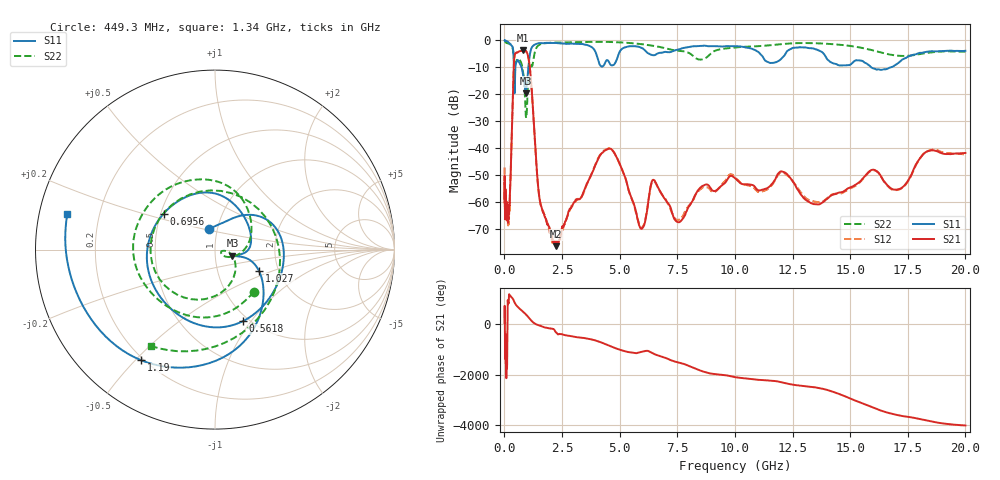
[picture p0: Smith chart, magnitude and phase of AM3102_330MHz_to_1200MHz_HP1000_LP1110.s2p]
! Date/Time: Tue, Sep 11, 2018 5:17 PM
! Network Analyzer: Agilent Technologies E8362B Rev: A.07.50.63
! Sweep from 0.010 to 20.000 GHz, 1601 Points, Sweep Type: LOG
! Power Supply: 4.949 V, 0.001 A
# Hz S DB R 50
!freq MagS11 AngS11 MagS21 AngS21 MagS12 AngS12 MagS22 AngS22
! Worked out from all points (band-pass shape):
!   1601 points, 10 MHz to 20 GHz, reference 50 ohm
!   highest |S21| = -3.57 dB at 813.7 MHz (marker M1); lowest = -76.5 dB at 2.249 GHz (marker M2)
!   |S21| within 3 dB of the highest: 429.5 MHz to 1.046 GHz (616.7 MHz wide, 83.6 % of centre)
!   lowest |S11| = -19.7 dB at 925.1 MHz (marker M3), VSWR 1.23, Z = 60.6 - j4.18 ohm
!   |S11| at or under -10 dB: 413.3 MHz to 476.9 MHz (63.61 MHz wide, 14.3 % of centre); 746.9 MHz to 1.041 GHz (294.2 MHz wide, 32.9 % of centre); 15.91 GHz to 16.77 GHz (858.9 MHz wide, 5.26 % of centre)
!   |S22| runs from -28.8 to -0.2 dB; largest |S21 - S12| = 0.0093
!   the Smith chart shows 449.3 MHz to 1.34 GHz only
!   S11 on the Smith chart (normalised r, x): 449.3 MHz: 0.91, +0.21; 561.8 MHz: 0.94, -0.91; 695.6 MHz: 0.52, +0.24; 1.027 GHz: 1.59, -0.41; 1.19 GHz: 0.19, -0.52; 1.34 GHz: 0.08, +0.12
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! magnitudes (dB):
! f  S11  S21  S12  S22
! 10 MHz  0.0  -51.9  -47.3  -0.3
! 35.55 MHz  0.0  -63.0  -63.6  -0.5
! 126.4 MHz  -0.4  -64.9  -65.4  -1.0
! 216.2 MHz  -1.0  -61.1  -63.7  -1.3
! 371.6 MHz  -2.9  -19.6  -19.7  -3.5
! 447.2 MHz  -19.1  -5.4  -5.5  -9.8
! 449.3 MHz  -18.6  -5.3  -5.4  -9.9
! 561.8 MHz  -7.4  -4.5  -4.5  -7.0
! 695.6 MHz  -9.1  -4.0  -4.0  -7.7
! 813.7 MHz  -13.1  -3.6  -3.7  -12.0
! 925.1 MHz  -19.7  -3.8  -3.9  -27.4
! 1.027 GHz  -11.3  -5.8  -5.8  -15.4
! 1.19 GHz  -2.6  -18.8  -18.8  -9.7
! 1.34 GHz  -1.4  -39.6  -40.0  -3.8
! 1.59 GHz  -1.0  -61.5  -61.5  -1.4
! 2.249 GHz  -1.0  -76.5  -75.9  -0.8
! 4.436 GHz  -7.4  -40.6  -40.5  -0.5
! 5.652 GHz  -2.2  -61.8  -62.1  -1.1
! 7.588 GHz  -3.3  -67.6  -66.7  -3.9
! 12.09 GHz  -6.2  -48.9  -49.1  -1.3
! 13.61 GHz  -3.6  -61.0  -60.2  -1.1
! 20 GHz  -3.9  -41.9  -42.4  -4.2
